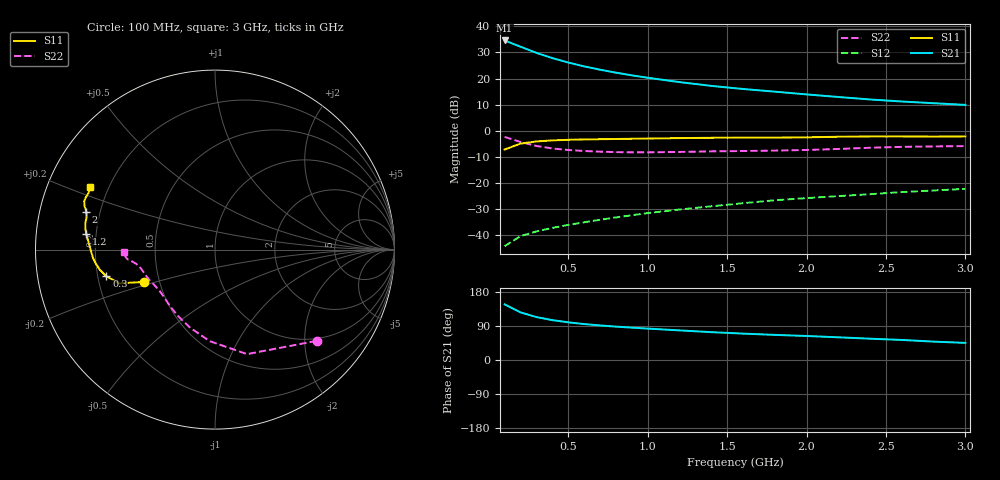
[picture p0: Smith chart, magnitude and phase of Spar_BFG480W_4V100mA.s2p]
! Filename: 4100BFG480.001
! Title: BFG480W
! Bias: Vce=4V; Ic=100mA
! Company: NXP Semiconductors NL
! User: Quality&Reliability T&D
! Measure time: 10 Nov 1999 / 12:04:01
#  MHz  S  MA  R 50
! Freq  S11  S21  S12  S22  :
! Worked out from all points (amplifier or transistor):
!   20 points, 100 MHz to 3 GHz, reference 50 ohm
!   highest |S21| = 34.6 dB at 100 MHz (marker M1)
!   |S21| within 3 dB of that: start of sweep to 225.8 MHz
!   unconditionally stable (mu >= 1): 717.5 MHz to end of sweep
!   at 400 MHz: K = 0.81, MSG = 32.5 dB, |S12| = -37.2 dB
!   at 1.2 GHz: K = 1.08, MAG = 22.7 dB, |S12| = -30.2 dB
!   at 3 GHz: K = 1.05, MAG = 14.8 dB, |S12| = -22.3 dB
!   S11 on the Smith chart (normalised r, x): 100 MHz: 0.41, -0.18; 300 MHz: 0.24, -0.11; 1.2 GHz: 0.16, +0.06; 2 GHz: 0.15, +0.14; 3 GHz: 0.13, +0.23
100  0.4361 -155.6  53.57 146.8  0.006144 68.9  0.7611 -41.9
200  0.5659 -160.6  40.67 125.6  0.009547 60.6  0.609 -73.0
300  0.6234 -166.2  31.03 113.3  0.01178 59.8  0.5109 -93.3
400  0.6525 -170.2  24.61 105.2  0.01374 61.3  0.4574 -107.4
500  0.6692 -173.4  20.26 99.4  0.01566 63.3  0.4273 -117.6
600  0.6809 -176.0  17.09 94.9  0.01762 65.3  0.4089 -125.2
700  0.6877 -178.3  14.77 91.2  0.01967 67.4  0.3972 -131.1
800  0.6941 179.7  12.95 88.1  0.02182 69.1  0.3895 -136.0
900  0.701 177.8  11.51 85.4  0.02402 70.9  0.3857 -140.3
1000  0.7082 176.1  10.35 82.9  0.02642 71.9  0.3853 -144.1
1200  0.7221 173.1  8.538 78.2  0.03094 73.5  0.392 -150.2
1400  0.732 170.8  7.226 73.5  0.03562 74.4  0.4022 -154.8
1600  0.7375 168.4  6.303 69.7  0.04088 75.3  0.4085 -158.2
1800  0.7376 165.9  5.603 66.3  0.04655 75.7  0.416 -161.9
2000  0.7472 163.6  4.959 63.4  0.0512 76.2  0.4278 -166.3
2200  0.7662 161.5  4.428 59.9  0.0559 76.3  0.4471 -169.9
2400  0.7766 159.8  3.968 56.2  0.06079 75.7  0.4716 -172.3
2600  0.7767 158.2  3.627 52.9  0.06689 75.0  0.4909 -173.7
2800  0.7721 155.9  3.364 48.5  0.07163 73.6  0.5003 -175.5
3000  0.7771 153.2  3.124 45.1  0.077 72.8  0.508 -178.4
